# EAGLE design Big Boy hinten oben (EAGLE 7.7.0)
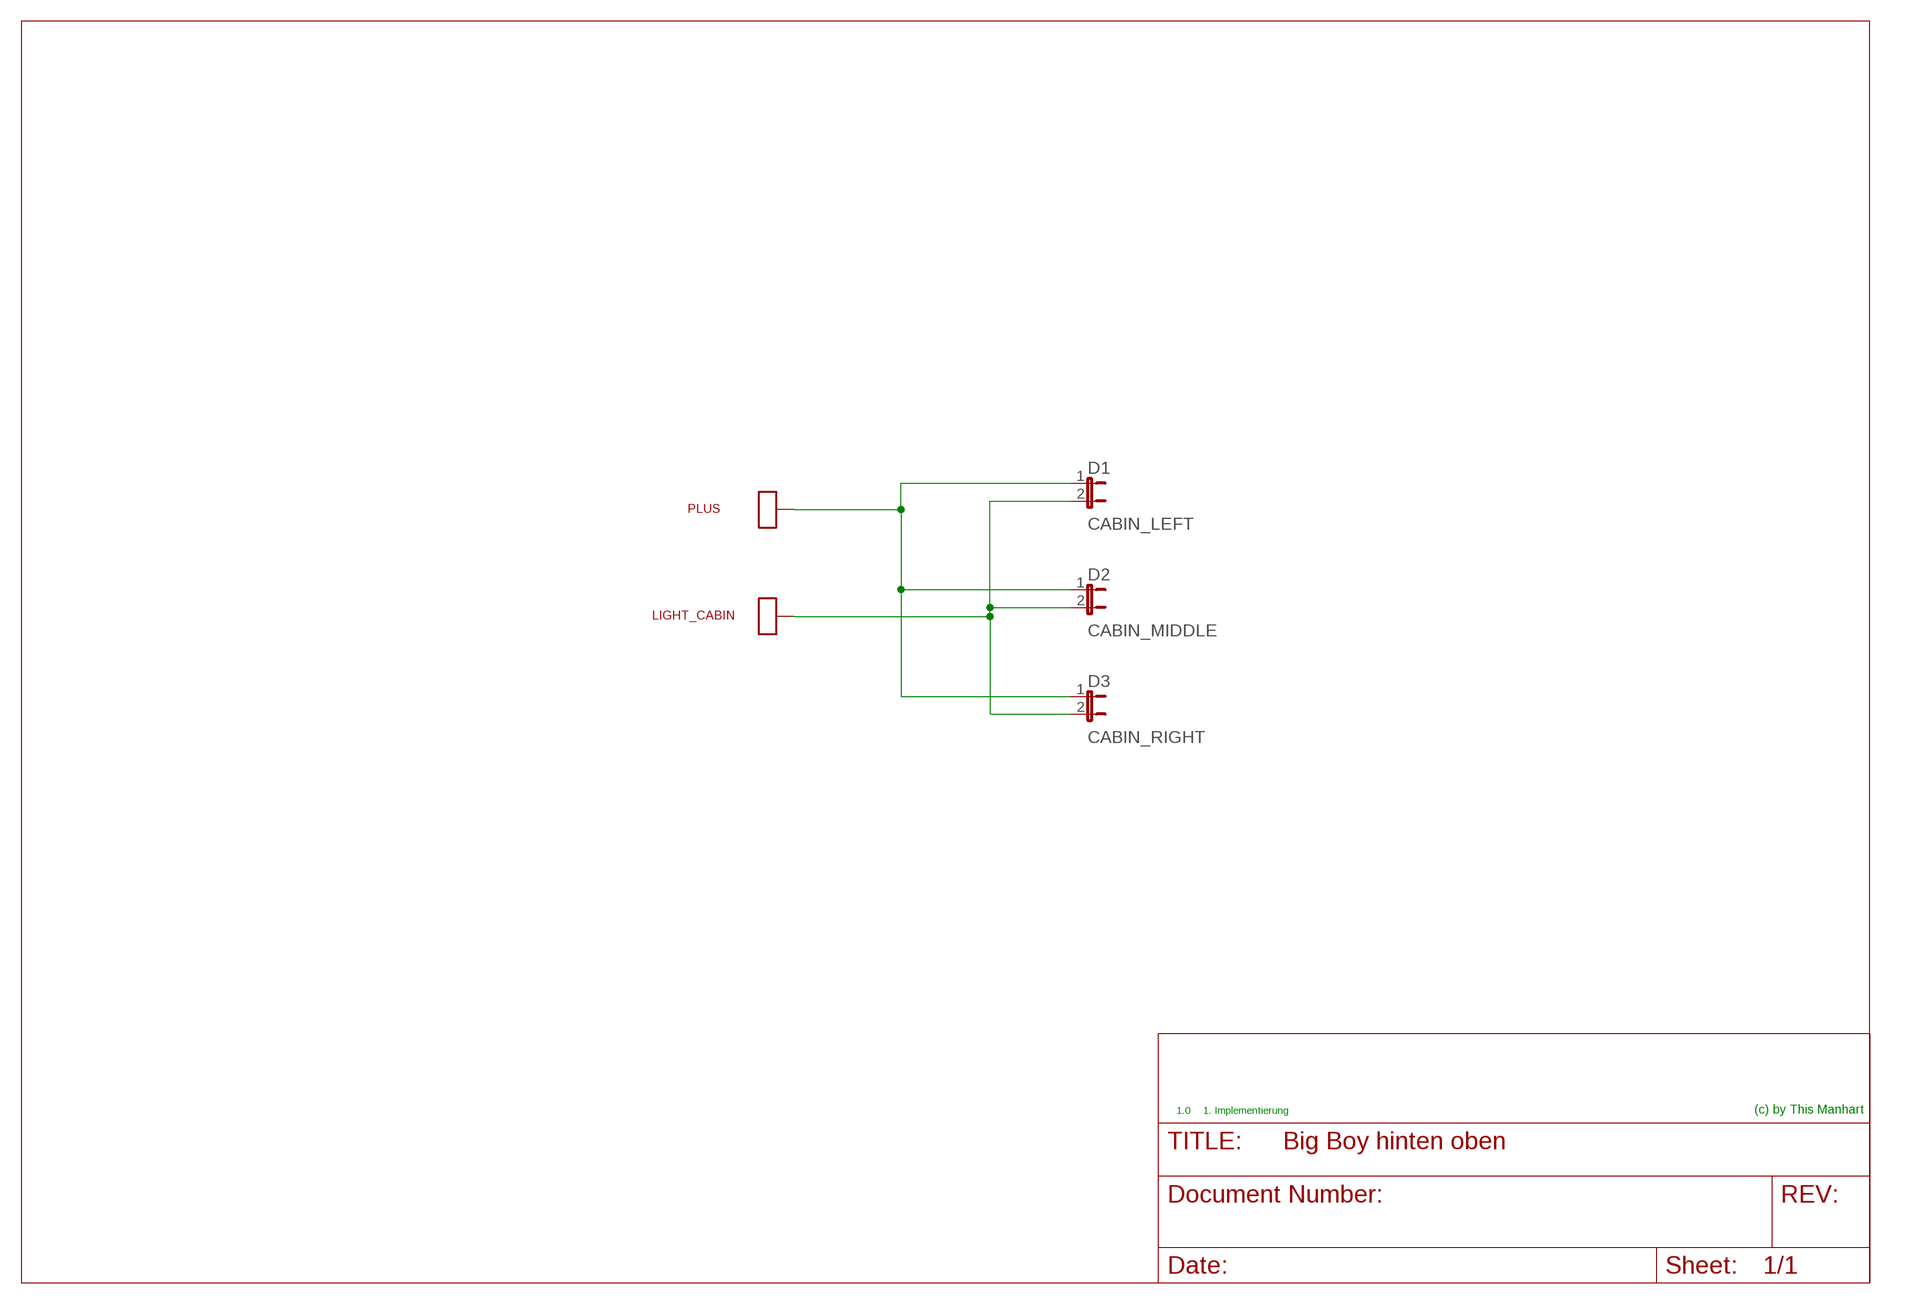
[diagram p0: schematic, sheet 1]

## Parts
D1  CABIN_LEFT  JUMPER_2P  [JUMPER_2P_2.54_OHNE]
D2  CABIN_MIDDLE  JUMPER_2P  [JUMPER_2P_2.54_OHNE]
D3  CABIN_RIGHT  JUMPER_2P  [JUMPER_2P_2.54_OHNE]
LIGHT_CABIN  SMD_LOETPAD  [SMD_LOETPAD_XL]
PLUS  SMD_LOETPAD  [SMD_LOETPAD_XL]

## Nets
N$1: D1.1 D2.1 D3.1 PLUS.P$1
N$2: D1.2 D2.2 D3.2 LIGHT_CABIN.P$1

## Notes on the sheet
- 1.0 | 1. Implementierung | (c) by This Manhart

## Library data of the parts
D1-D3 = 0_mm:JUMPER_2P
LIGHT_CABIN PLUS = 0_mm:SMD_LOETPAD

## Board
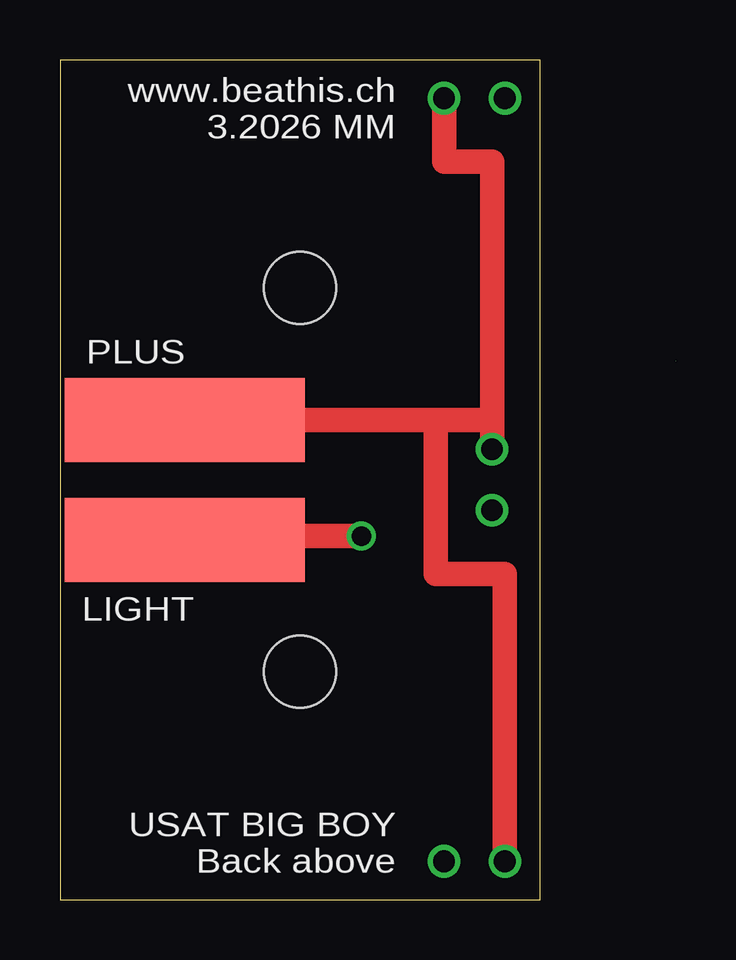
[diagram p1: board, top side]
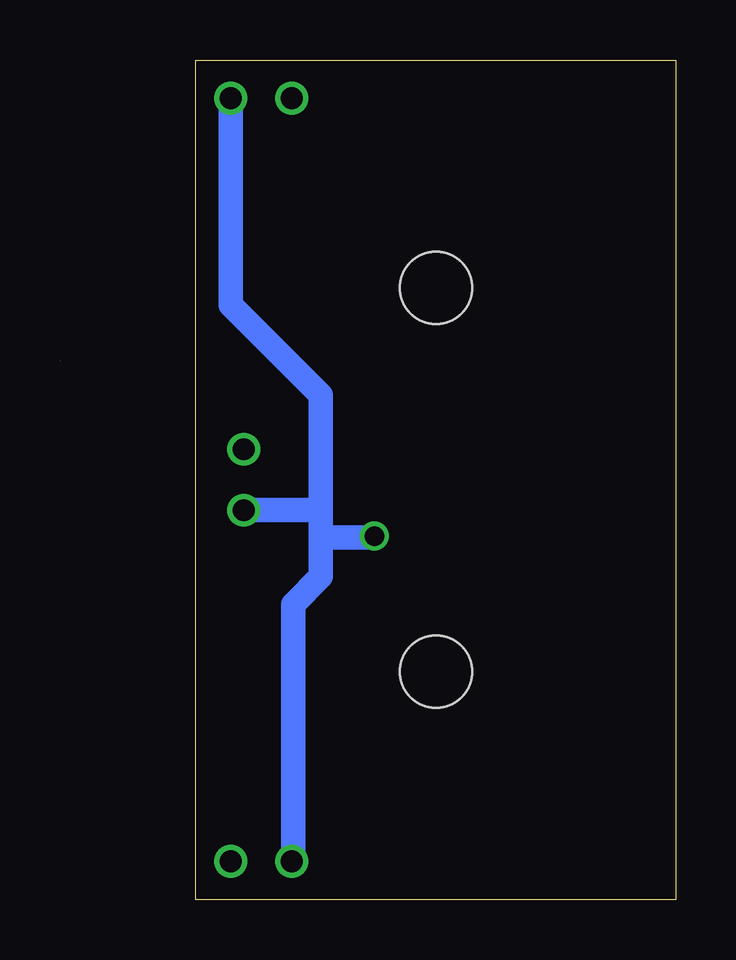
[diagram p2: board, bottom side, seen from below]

Size 25.66 x 35 mm. Coordinates in mm from the lower left corner, seen from the top.
Outline: 25.65,22.45 25.66,22.45
Outline: 20,0 20,35 0,35 0,0 20,0
Copper layers (1*16): Top 0.035mm / dielectric 1.5mm / Bottom 0.035mm
Design rules "pcb-pool": minimum track width 6mil, minimum drill 12mil, track to track 6mil, track to pad 6mil, pad to pad 6mil, via to via 6mil, smd to smd 8mil, copper to edge 40mil, drill to drill 20mil, minimum pad ring 8mil, minimum via ring 8mil, stop-mask expansion 6mil, vias tented up to drill 0mil, thermal gap 10mil
Holes 3 mm at 10,9.5 10,25.5

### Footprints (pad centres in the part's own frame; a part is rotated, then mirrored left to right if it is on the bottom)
JUMPER_2P_2.54_OHNE = drill 0.914: 1 -2.54,0; 2 0,0
SMD_LOETPAD_XL = smd 10 x 3.5: P$1 0,0

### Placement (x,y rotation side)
D1  18.54,33.4 0 top
D2  18,16.23 270 top
D3  16,1.6 180 top
LIGHT_CABIN  5.2,15 0 top
PLUS  5.2,20 180 top

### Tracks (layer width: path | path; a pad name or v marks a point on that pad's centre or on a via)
N$1
  Top 1.016: PLUS.P$1 15.65,20 | 15.65,20 18,20 D2.1 18,30.76 16,30.76 D1.1 | D3.1 18.54,13.58 15.65,13.58 15.65,20
N$2  (via drill 0.8 pad 1.2)
  Top 1.016: LIGHT_CABIN.P$1 5.2,15.15 v12.56,15.15
  Bottom 1.016: D1.2 18.54,24.78 14.79,21.03 14.79,16.23 | D3.2 15.95,1.65 15.95,12.31 14.79,13.47 14.79,15.1 | 14.79,15.1 14.79,16.23 | 14.79,16.23 D2.2 | v12.56,15.15 12.56,15.1 14.79,15.1

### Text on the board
tNames: www.beathis.ch / 3.2026 MM | PLUS | LIGHT | USAT BIG BOY / Back above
